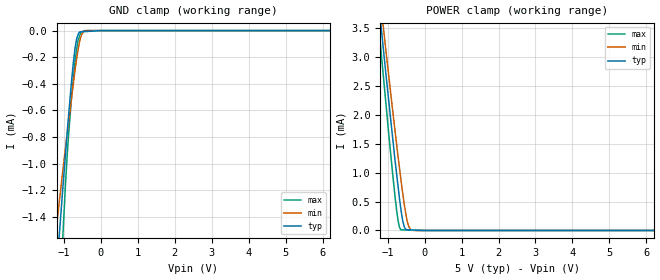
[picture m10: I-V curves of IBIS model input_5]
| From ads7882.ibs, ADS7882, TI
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|   input_5 Model
[Model]   input_5
Model_type   Input
Vinl = 0.8
Vinh = 4
|   typ   min   max
|   (nom PVT)   (Fast PVT)   (slow PVT)
|C_comp from frequency sweep method (F=1.5MHz)
|Average
C_comp   2.321e-12   2.259e-12   2.384e-12
|C_comp from LC tank measurement(L=1nH)
|Resonant Frequency(Hz)   3.590e+09   3.630e+09   3.530e+09
|C_comp   1.967e-12   1.924e-12   2.035e-12
| Where nom  PVT is Nominal Process,  5V,  25C
|   Fast PVT is Strong Process,   5.25V,  -40C
|   Slow PVT is Weak Process,   4.75V,  85C
[Model Spec]
Vinh   4   3.75   4.25
[Voltage Range]   5   4.75   5.25
|Ambient Temperature   25   85   -40
|Junction Temperature
[Temperature Range]   25   85   -40
[Power Clamp Reference]   5   4.75   5.25
[GND Clamp Reference]   0   0   0
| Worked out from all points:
|   GND clamp passes 1 mA (typ) near -0.98 V on its own axis
|   POWER clamp passes 1 mA (typ) near -0.76 V on its own axis
[GND Clamp]
|   Voltage   I(typ)   I(min)   I(max)
-5V       -16.61mA   -11.2mA    -29.34mA
-1.246V   -1.986mA   -1.585mA   -2.912mA
-1.125V   -1.54mA    -1.289mA   -2.133mA
-1.025V   -1.168mA   -1.043mA   -1.524mA
-905mV    -743.8uA   -756.5uA   -911.3uA
-800mV    -399.4uA   -522.2uA   -521.7uA
-690mV    -116.1uA   -278.5uA   -208.2uA
-621.5mV  -35.9uA    -152.2uA   -78.33uA
-575mV    -10.26uA   -81.89uA   -39.65uA
-468.5mV  -8.361uA   -7.771uA   -3.795uA
-373.5mV  -6.666uA   0A         0A
10V       0A         0A         0A
[POWER Clamp]
|   Voltage   I(typ)   I(min)   I(max)
-5V       28.42mA    26.79mA    30.51mA
-1.246V   3.957mA    4.265mA    3.562mA
-1.029V   2.594mA    3.007mA    2.071mA
-873.5mV  1.652mA    2.126mA    1.035mA
-752.8mV  950.3uA    1.463mA    326.2uA
-710.7mV  719.5uA    1.238mA    142uA
-642.5mV  372uA      886.8uA    10.9uA
-550mV    61.52uA    450.3uA    8.814uA
-478mV    12.85uA    179.4uA    7.189uA
-378.2mV  10.17uA    16.2uA     4.937uA
-278.5mV  7.487uA    20.47nA    2.686uA
10V       0A         0A         0A
